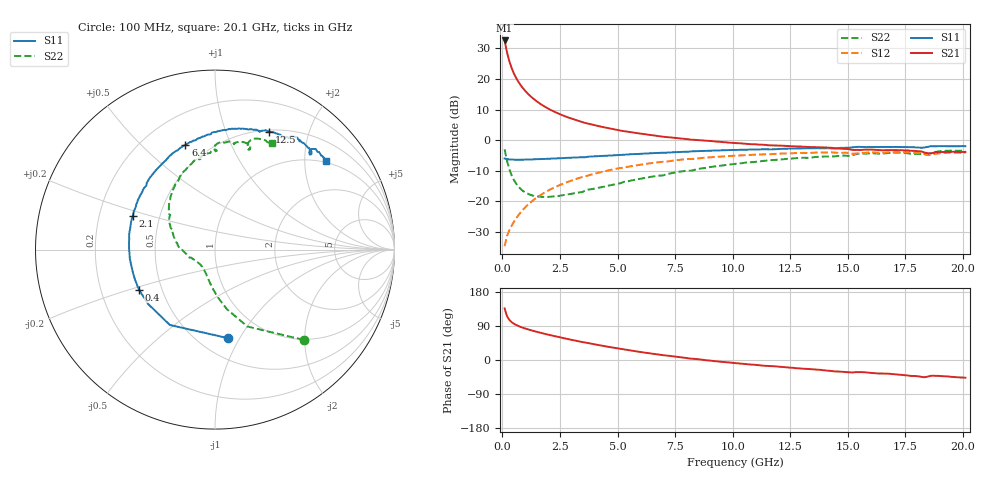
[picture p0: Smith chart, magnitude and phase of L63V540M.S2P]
!  Infineon Technologies AG
! BFR380L3 , PF131585-7, No.6, Th 09.10.01, soldered on pcb-board, measured with PP GSG850
!  Vce=3.5 V,  Ic=40.0 mA
! Common Emitter S-Parameters:  15. November 2001
#  GHz  S  MA  R  50
! f  S11  S21  S12  S22
! GHz  Mag  Ang  Mag  Ang  Mag  Ang  Mag  Ang
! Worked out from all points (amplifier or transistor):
!   201 points, 100 MHz to 20.1 GHz, reference 50 ohm
!   highest |S21| = 32.6 dB at 100 MHz (marker M1)
!   |S21| within 3 dB of that: start of sweep to 179.5 MHz
!   unconditionally stable (mu >= 1): 1.072 GHz to 4.323 GHz
!   at 3.4 GHz: K = 1.02, MAG = 8.4 dB, |S12| = -12.3 dB
!   at 10.1 GHz: K = 0.96, MSG = 2.1 dB, |S12| = -5.1 dB
!   at 20.1 GHz: K = 0.99, MSG = 0.1 dB, |S12| = -4.1 dB
!   S11 on the Smith chart (normalised r, x): 100 MHz: 0.68, -0.90; 400 MHz: 0.37, -0.21; 2.1 GHz: 0.35, +0.17; 6.4 GHz: 0.37, +0.69; 12.5 GHz: 0.52, +1.42; 20.1 GHz: 0.95, +2.53
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0.1  0.4991 -81.5  42.78 136.3  0.01828 64.3  0.7063 -45.4
0.2  0.4895 -120.9  27.7 116.0  0.02671 57.4  0.465 -67.2
0.3  0.4802 -140.7  19.8 106.2  0.03297 58.5  0.3382 -78.7
0.4  0.479 -152.2  15.28 100.1  0.03918 60.7  0.267 -86.5
0.5  0.476 -159.8  12.39 95.7  0.04558 63.1  0.2226 -92.5
0.6  0.4748 -165.5  10.41 92.5  0.0523 64.7  0.1933 -97.5
0.7  0.475 -170.1  8.974 89.6  0.05873 66.1  0.1727 -101.9
0.9  0.4768 -177.1  7.031 85.0  0.07271 67.5  0.1463 -109.3
1.1  0.4795 177.4  5.793 81.1  0.08659 68.0  0.1326 -116.1
1.4  0.4851 170.6  4.585 75.9  0.1077 67.8  0.1212 -124.3
1.7  0.4884 164.8  3.804 71.1  0.1286 67.0  0.1173 -131.7
2.1  0.4943 158.0  3.115 65.3  0.1564 65.2  0.1184 -139.9
2.7  0.5076 148.6  2.471 57.2  0.1972 61.9  0.1261 -151.0
3.5  0.5235 137.4  1.955 47.1  0.2504 56.7  0.1422 -161.8
4.9  0.5633 121.1  1.488 31.6  0.3359 47.1  0.1883 178.1
6.4  0.6055 105.8  1.215 17.4  0.4162 36.6  0.2486 160.1
6.8  0.6153 102.2  1.16 14.1  0.4349 33.6  0.261 155.4
10.1  0.6878 77.9  0.893 -8.1  0.5537 12.0  0.407 125.2
12.5  0.7225 65.5  0.7935 -20.2  0.6094 -2.7  0.4964 105.3
13.5  0.7341 60.7  0.7662 -24.7  0.6199 -8.6  0.5222 98.6
16.8  0.7696 48.4  0.6825 -36.2  0.628 -24.5  0.6136 77.8
20.1  0.7918 38.7  0.6371 -46.7  0.6223 -38.3  0.6723 61.8
